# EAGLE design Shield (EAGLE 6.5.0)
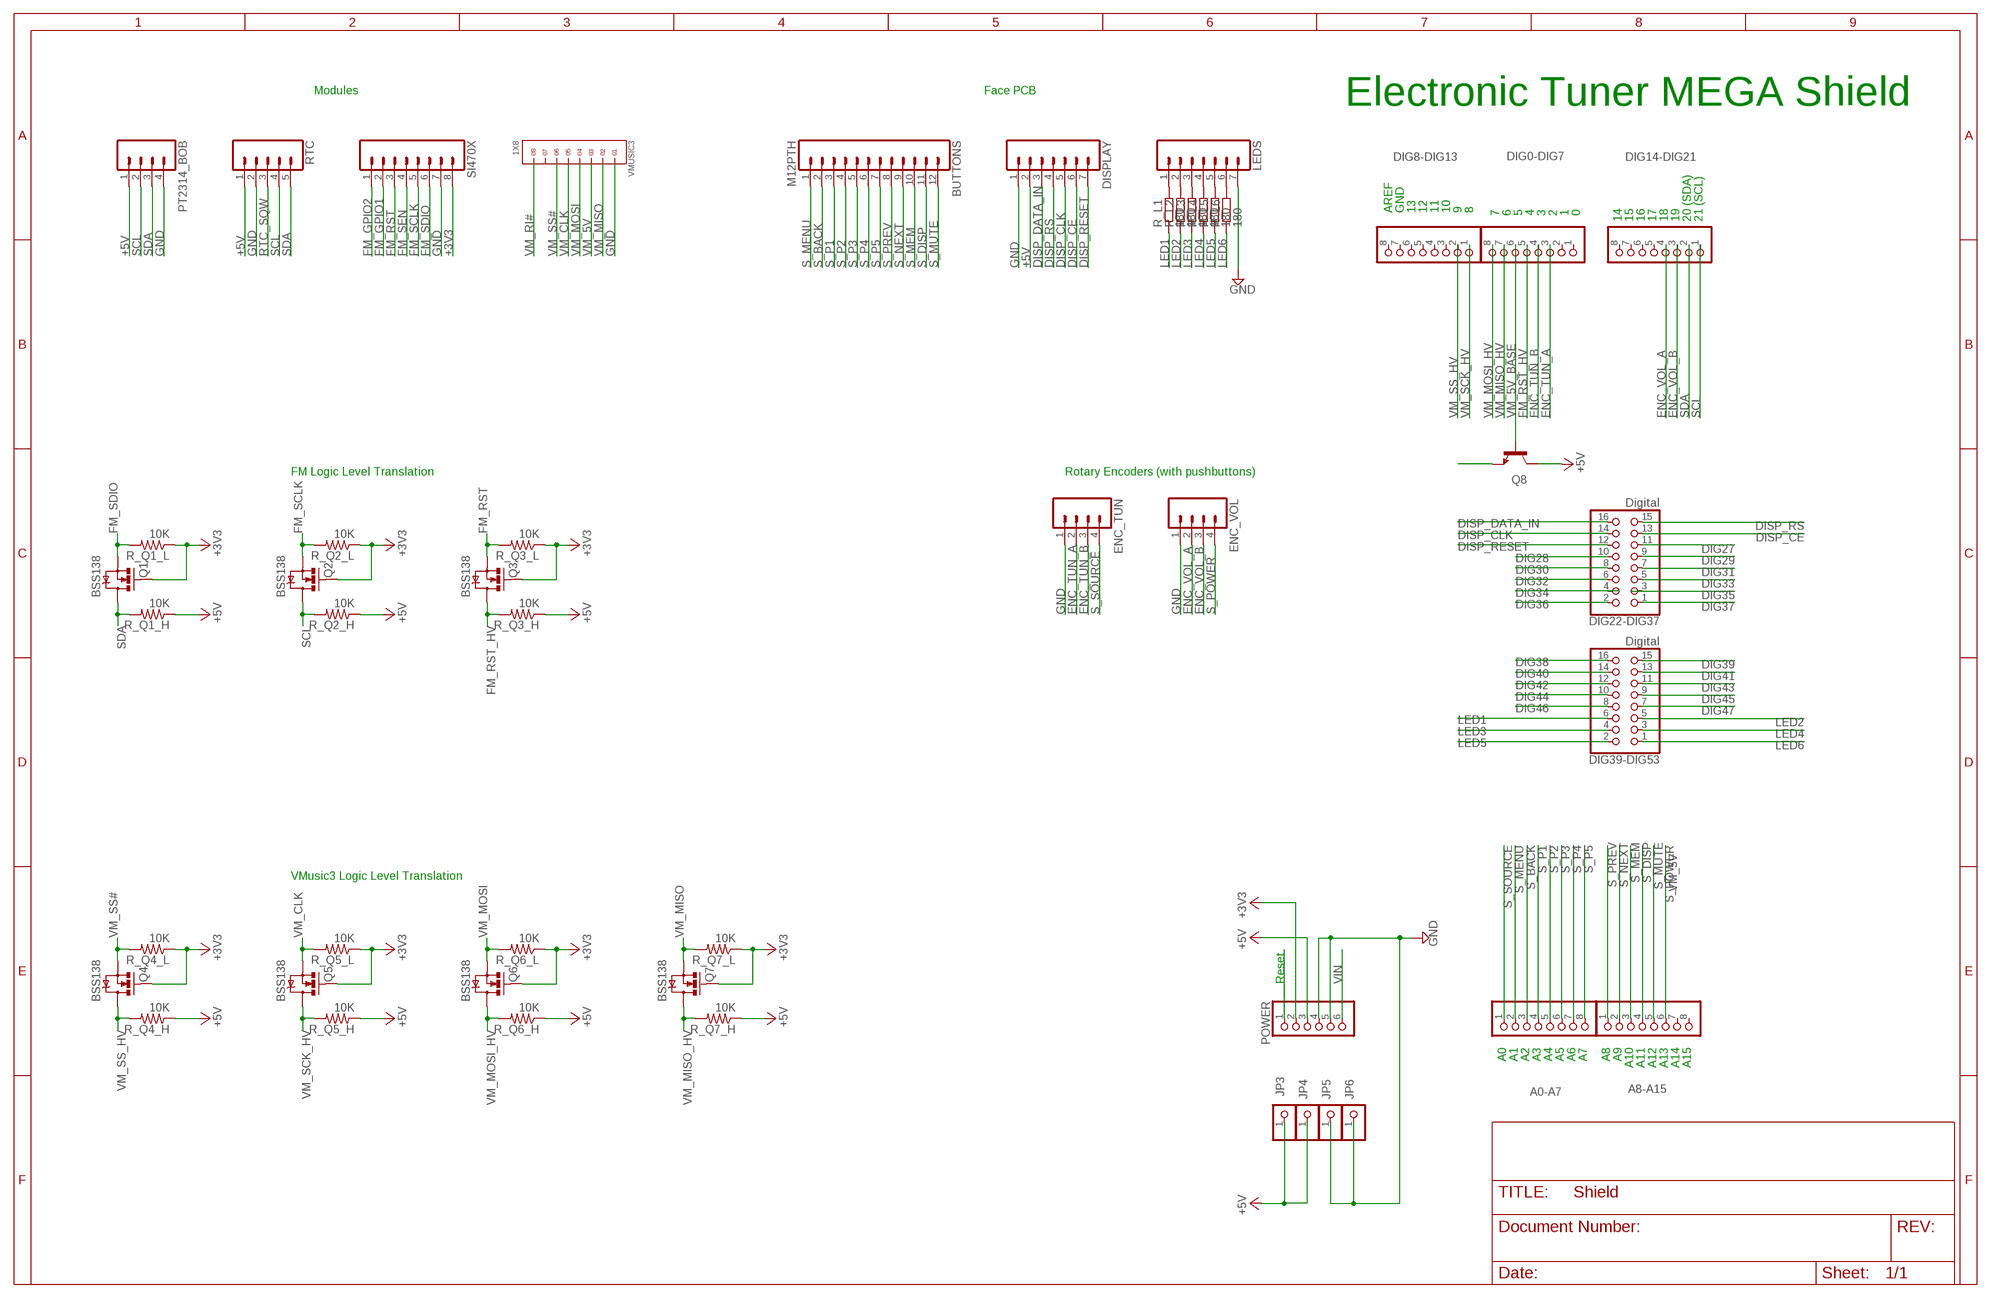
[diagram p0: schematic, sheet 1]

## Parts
A0-A7  PINHD-1X8  [1X08]
A8-A15  PINHD-1X8  [1X08]
BUTTONS  M12PTH  [1X12]
DIG0-DIG7  PINHD-1X8  [1X08]
DIG8-DIG13  PINHD-1X8  [1X08]
DIG14-DIG21  PINHD-1X8  [1X08]
DIG22-DIG37  Digital  PINHD-2X8  [2X08]
DIG39-DIG53  Digital  PINHD-2X8  [2X08]
DISPLAY  M07  [1X07]
ENC_TUN  M04PTH  [1X04]
ENC_VOL  M04PTH  [1X04]
JP3  PINHD-1X1  [1X01]
JP4  PINHD-1X1  [1X01]
JP5  PINHD-1X1  [1X01]
JP6  PINHD-1X1  [1X01]
LEDS  M07  [1X07]
POWER  PINHD-1X6  [1X06]
PT2314_BOB  M04PTH  [1X04]
Q1  BSS138  MOSFET-NCHANNELSMD  [SOT23-3]
Q2  BSS138  MOSFET-NCHANNELSMD  [SOT23-3]
Q3  BSS138  MOSFET-NCHANNELSMD  [SOT23-3]
Q4  BSS138  MOSFET-NCHANNELSMD  [SOT23-3]
Q5  BSS138  MOSFET-NCHANNELSMD  [SOT23-3]
Q6  BSS138  MOSFET-NCHANNELSMD  [SOT23-3]
Q7  BSS138  MOSFET-NCHANNELSMD  [SOT23-3]
Q8  BC848ALT1SMD  [SOT23]
R_L1  180  R-EU_R0603  [R0603]
R_L2  180  R-EU_R0603  [R0603]
R_L3  180  R-EU_R0603  [R0603]
R_L4  180  R-EU_R0603  [R0603]
R_L5  180  R-EU_R0603  [R0603]
R_L6  180  R-EU_R0603  [R0603]
R_Q1_H  10K  RESISTOR0603-RES  [0603-RES]
R_Q1_L  10K  RESISTOR0603-RES  [0603-RES]
R_Q2_H  10K  RESISTOR0603-RES  [0603-RES]
R_Q2_L  10K  RESISTOR0603-RES  [0603-RES]
R_Q3_H  10K  RESISTOR0603-RES  [0603-RES]
R_Q3_L  10K  RESISTOR0603-RES  [0603-RES]
R_Q4_H  10K  RESISTOR0603-RES  [0603-RES]
R_Q4_L  10K  RESISTOR0603-RES  [0603-RES]
R_Q5_H  10K  RESISTOR0603-RES  [0603-RES]
R_Q5_L  10K  RESISTOR0603-RES  [0603-RES]
R_Q6_H  10K  RESISTOR0603-RES  [0603-RES]
R_Q6_L  10K  RESISTOR0603-RES  [0603-RES]
R_Q7_H  10K  RESISTOR0603-RES  [0603-RES]
R_Q7_L  10K  RESISTOR0603-RES  [0603-RES]
RTC  M05PTH  [1X05]
SI470X  M081X08  [1X08]
VMUSIC3  1X8  [1X8]

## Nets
+3V3 [power]: POWER.2 Q1.1(G) Q2.1(G) Q3.1(G) Q4.1(G) Q5.1(G) Q6.1(G) Q7.1(G) R_Q1_L.1 R_Q2_L.1 R_Q3_L.1 R_Q4_L.1 R_Q5_L.1 R_Q6_L.1 R_Q7_L.1 SI470X.8
+5V [power]: DISPLAY.2 JP3.1 JP4.1 POWER.3 PT2314_BOB.1 Q8.3(C) R_Q1_H.1 R_Q2_H.1 R_Q3_H.1 R_Q4_H.1 R_Q5_H.1 R_Q6_H.1 R_Q7_H.1 RTC.1
DIG27: DIG22-DIG37.11
DIG28: DIG22-DIG37.10
DIG29: DIG22-DIG37.9
DIG30: DIG22-DIG37.8
DIG31: DIG22-DIG37.7
DIG32: DIG22-DIG37.6
DIG33: DIG22-DIG37.5
DIG36: DIG22-DIG37.2
DIG37: DIG22-DIG37.1
DIG38: DIG39-DIG53.16
DIG39: DIG39-DIG53.15
DIG40: DIG39-DIG53.14
DIG41: DIG39-DIG53.13
DIG42: DIG39-DIG53.12
DIG43: DIG39-DIG53.11
DIG44: DIG39-DIG53.10
DIG45: DIG39-DIG53.9
DIG46: DIG39-DIG53.8
DIG47: DIG39-DIG53.7
DISP_CE: DIG22-DIG37.13 DISPLAY.6
DISP_CLK: DIG22-DIG37.14 DISPLAY.5
DISP_DATA_IN: DIG22-DIG37.16 DISPLAY.3
DISP_RESET: DIG22-DIG37.12 DISPLAY.7
DISP_RS: DIG22-DIG37.15 DISPLAY.4
ENC_TUN_A: DIG0-DIG7.3 ENC_TUN.2
ENC_TUN_B: DIG0-DIG7.4 ENC_TUN.3
ENC_VOL_A: DIG14-DIG21.4 ENC_VOL.2
ENC_VOL_B: DIG14-DIG21.3 ENC_VOL.3
FM_GPIO1: SI470X.2
FM_GPIO2: SI470X.1
FM_RST: Q3.2(S) R_Q3_L.2 SI470X.3
FM_RST_HV: DIG0-DIG7.5 Q3.3(D) R_Q3_H.2
FM_SCLK: Q2.2(S) R_Q2_L.2 SI470X.5
FM_SDIO: Q1.2(S) R_Q1_L.2 SI470X.6
FM_SEN: SI470X.4
GND [gnd]: DISPLAY.1 ENC_TUN.1 ENC_VOL.1 JP5.1 JP6.1 LEDS.7 POWER.4 POWER.5 PT2314_BOB.4 RTC.2 SI470X.7 VMUSIC3.1
LED1: DIG39-DIG53.6 R_L1.1
LED2: DIG39-DIG53.5 R_L2.1
LED3: DIG39-DIG53.4 R_L3.1
LED4: DIG39-DIG53.3 R_L4.1
LED5: DIG39-DIG53.2 R_L5.1
LED6: DIG39-DIG53.1 R_L6.1
N$13: LEDS.1 R_L1.2
N$14: LEDS.2 R_L2.2
N$15: LEDS.3 R_L3.2
N$16: LEDS.4 R_L4.2
N$17: LEDS.5 R_L5.2
N$18: LEDS.6 R_L6.2
RESET: POWER.1
RTC_SQW: RTC.3
S_BACK: A0-A7.3 BUTTONS.2
S_DISP: A8-A15.4 BUTTONS.11
S_MEM: A8-A15.3 BUTTONS.10
S_MENU: A0-A7.2 BUTTONS.1
S_MUTE: A8-A15.5 BUTTONS.12
S_NEXT: A8-A15.2 BUTTONS.9
S_P1: A0-A7.4 BUTTONS.3
S_P2: A0-A7.5 BUTTONS.4
S_P3: A0-A7.6 BUTTONS.5
S_P4: A0-A7.7 BUTTONS.6
S_P5: A0-A7.8 BUTTONS.7
S_POWER: A8-A15.6 ENC_VOL.4
S_PREV: A8-A15.1 BUTTONS.8
S_SOURCE: A0-A7.1 ENC_TUN.4
SCL: DIG14-DIG21.1 PT2314_BOB.2 Q2.3(D) R_Q2_H.2 RTC.4
SDA: DIG14-DIG21.2 PT2314_BOB.3 Q1.3(D) R_Q1_H.2 RTC.5
VIN [power]: POWER.6
VM_5V [power]: Q8.2(E) VMUSIC3.3
VM_5V_BASE: DIG0-DIG7.6 Q8.1(B)
VM_CLK: Q5.2(S) R_Q5_L.2 VMUSIC3.5
VM_MISO: Q7.2(S) R_Q7_L.2 VMUSIC3.2
VM_MISO_HV: DIG0-DIG7.7 Q7.3(D) R_Q7_H.2
VM_MOSI: Q6.2(S) R_Q6_L.2 VMUSIC3.4
VM_MOSI_HV: DIG0-DIG7.8 Q6.3(D) R_Q6_H.2
VM_RI#: VMUSIC3.8
VM_SCK_HV: DIG8-DIG13.1 Q5.3(D) R_Q5_H.2
VM_SS#: Q4.2(S) R_Q4_L.2 VMUSIC3.6
VM_SS_HV: DIG8-DIG13.2 Q4.3(D) R_Q4_H.2
Unconnected: A8-A15.7 A8-A15.8 DIG0-DIG7.1 DIG0-DIG7.2 DIG8-DIG13.3 DIG8-DIG13.4 DIG8-DIG13.5 DIG8-DIG13.6 DIG8-DIG13.7 DIG8-DIG13.8 DIG14-DIG21.5 DIG14-DIG21.6 DIG14-DIG21.7 DIG14-DIG21.8 DIG22-DIG37.3 DIG22-DIG37.4 VMUSIC3.7

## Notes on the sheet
- Modules | Face PCB
- Electronic Tuner MEGA Shield
- AREF | GND | 13 | 12 | 11 | 10 | 9 | 8 | 7 | 6 | 5 | 4 | 3 | 2 | 1 | 0
- 14 | 15 | 16 | 17 | 18 | 19 | 20 (SDA) | 21 (SCL)
- FM Logic Level Translation | Rotary Encoders (with pushbuttons)
- VMusic3 Logic Level Translation
- Reset
- A0 | A1 | A2 | A3 | A4 | A5 | A6 | A7 | A8 | A9 | A10 | A11 | A12 | A13 | A14 | A15

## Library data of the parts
A0-A7 A8-A15 DIG0-DIG7 DIG8-DIG13 DIG14-DIG21 = pinhead:PINHD-1X8: PIN HEADER
BUTTONS = SparkFun-Connectors:M12: Header 12 Standard 12-pin 0.1" header. Use with straight break away headers (SKU : PRT-00116), right angle break away headers (PRT-00553), swiss pins (PRT-00743), machine pins (PRT-00117), and female headers (PRT-00115).
DIG22-DIG37 DIG39-DIG53 = pinhead:PINHD-2X8: PIN HEADER
DISPLAY LEDS = SparkFun-Connectors:M07: Header 7 Standard 7-pin 0.1" header. Use with straight break away headers (SKU : PRT-00116), right angle break away headers (PRT-00553), swiss pins (PRT-00743), machine pins (PRT-00117), and female headers (PRT-00115). NOTES ON THE VARIANTS LOCK and LOCK_LONGPADS... This footprint was designed to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
ENC_TUN ENC_VOL PT2314_BOB = SparkFun-Connectors:M04: Header 4 Standard 4-pin 0.1" header. Use with straight break away headers (SKU : PRT-00116), right angle break away headers (PRT-00553), swiss pins (PRT-00743), machine pins (PRT-00117), and female headers (PRT-00115). Molex polarized connector foot print use with SKU : PRT-08231 with associated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
JP3-JP6 = pinhead:PINHD-1X1: PIN HEADER
POWER = pinhead:PINHD-1X6: PIN HEADER
Q1-Q7 = SparkFun:MOSFET-NCHANNEL
Q8 = transistor-npn:BC848*: NPN Transistor
R_L1-R_L6 = resistor:R-EU_: RESISTOR, European symbol
R_Q1_H R_Q1_L R_Q2_H R_Q2_L R_Q3_H R_Q3_L R_Q4_H R_Q4_L R_Q5_H R_Q5_L R_Q6_H R_Q6_L R_Q7_H R_Q7_L = SparkFun:RESISTOR: Resistor
RTC = SparkFun-Connectors:M05: Header 5 Standard 5-pin 0.1" header. Use with straight break away headers (SKU : PRT-00116), right angle break away headers (PRT-00553), swiss pins (PRT-00743), machine pins (PRT-00117), and female headers (PRT-00115). Molex polarized connector foot print use with SKU : PRT-08230 with associated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
SI470X = SparkFun-Connectors:M08: Header 8 Standard 8-pin 0.1" header. Use with straight break away headers (SKU : PRT-00116), right angle break away headers (PRT-00553), swiss pins (PRT-00743), machine pins (PRT-00117), and female headers (PRT-00115).
VMUSIC3 = headers(2mm):1X8

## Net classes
0 default: width 0.203 mm, drill 0.406 mm, clearance 0.203 mm
1 power: width 0.61 mm, drill 0.711 mm, clearance 0.203 mm
2 gnd: width 0.305 mm, drill 0.711 mm, clearance 0.203 mm
3 usbvcc: width 0.508 mm, drill 0.711 mm, clearance 0.203 mm

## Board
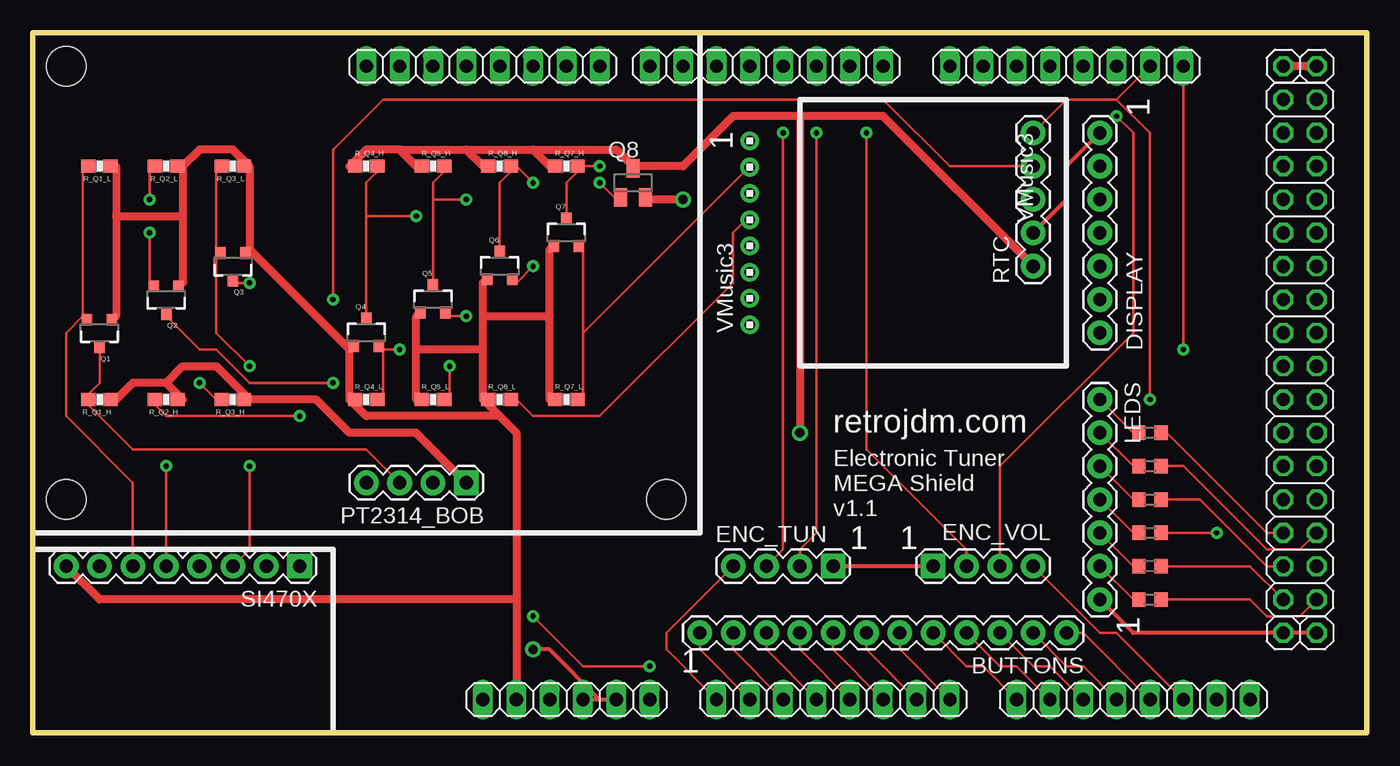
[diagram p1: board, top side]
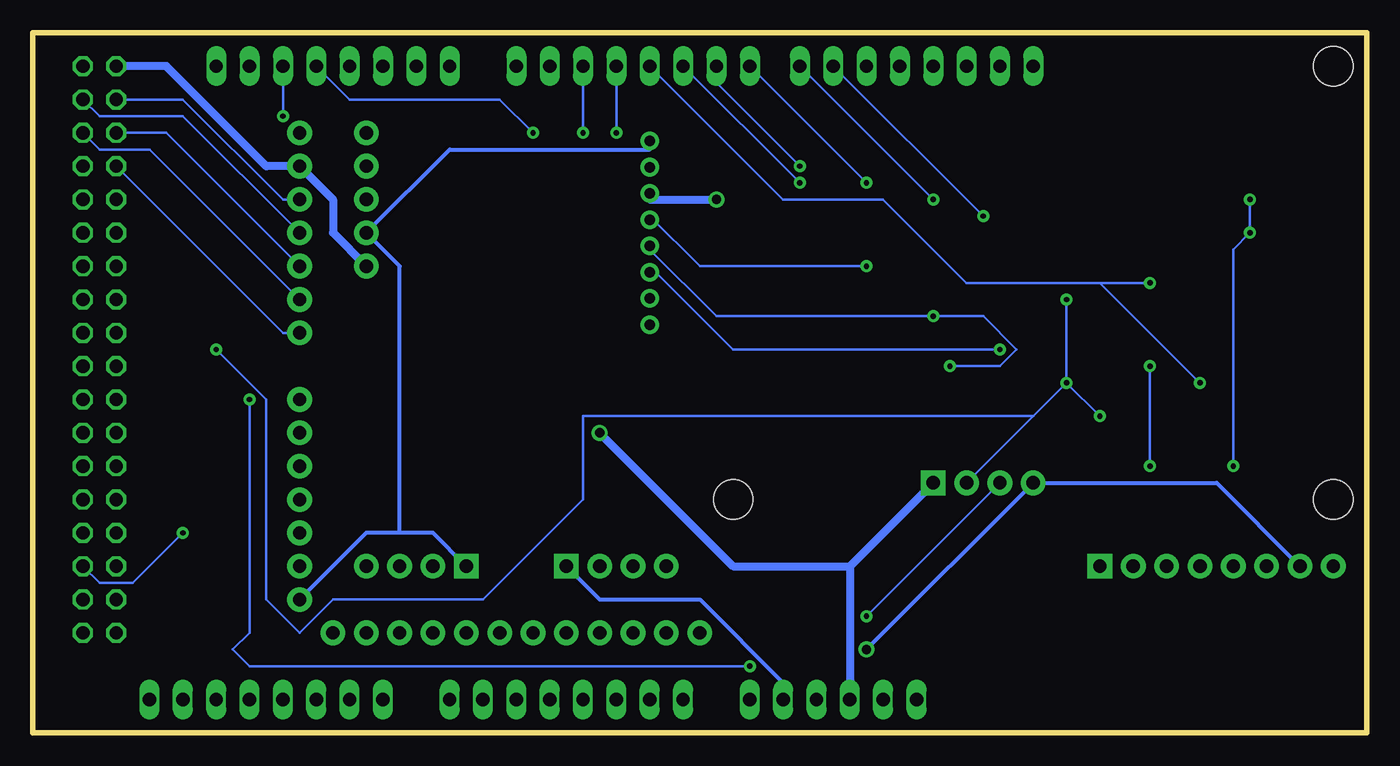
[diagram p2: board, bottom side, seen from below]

Size 101.6 x 53.34 mm. Coordinates in mm from the lower left corner, seen from the top.
Outline: 101.6,53.34 0,53.34 0,0 101.6,0 101.6,53.34
Copper layers (1*16): Top 0.035mm / dielectric 1.5mm / Bottom 0.035mm
Design rules "default *": minimum track width 8mil, minimum drill 16mil, track to track 10mil, track to pad 15mil, pad to pad 15mil, via to via 10mil, smd to smd 10mil, copper to edge 40mil, drill to drill 10mil, minimum pad ring 10mil, minimum via ring 10mil, stop-mask expansion 4mil, vias tented up to drill 0mil, thermal gap 10mil
Holes 3 mm at 48.26,17.78 2.54,17.78 2.54,50.8

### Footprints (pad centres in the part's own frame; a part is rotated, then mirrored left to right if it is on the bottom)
1X08 = drill 1.016 long: 1 -8.89,0; 2 -6.35,0; 3 -3.81,0; 4 -1.27,0; 5 1.27,0; 6 3.81,0; 7 6.35,0; 8 8.89,0
1X12 = drill 1.016 pad 1.88: 1 0,0; 2 2.54,0; 3 5.08,0; 4 7.62,0; 5 10.16,0; 6 12.7,0; 7 15.24,0; 8 17.78,0; 9 20.32,0; 10 22.86,0; 11 25.4,0; 12 27.94,0
2X08 = drill 1.016 octagon: 1 -8.89,-1.27; 2 -8.89,1.27; 3 -6.35,-1.27; 4 -6.35,1.27; 5 -3.81,-1.27; 6 -3.81,1.27; 7 -1.27,-1.27; 8 -1.27,1.27; 9 1.27,-1.27; 10 1.27,1.27; 11 3.81,-1.27; 12 3.81,1.27; 13 6.35,-1.27; 14 6.35,1.27; 15 8.89,-1.27; 16 8.89,1.27
1X07 = drill 1.016 pad 1.88: 1 0,0; 2 2.54,0; 3 5.08,0; 4 7.62,0; 5 10.16,0; 6 12.7,0; 7 15.24,0
1X04 = drill 1.016 pad 1.88 square: 1 0,0 | drill 1.016 pad 1.88: 2 2.54,0; 3 5.08,0; 4 7.62,0
1X01 = drill 1.016 octagon: 1 0,0
1X06 = drill 1.016 long: 1 -6.35,0; 2 -3.81,0; 3 -1.27,0; 4 1.27,0; 5 3.81,0; 6 6.35,0
SOT23-3 = smd 0.8 x 0.9: 1 -0.95,-1; 2 0.95,-1; 3 0,1.1
SOT23 = smd 1 x 1.4: 1 -0.95,-1.1; 2 0.95,-1.1; 3 0,1.1
R0603 = smd 1 x 1.1: 1 -0.85,0; 2 0.85,0
0603-RES = smd 1.1 x 1: 1 -0.85,0; 2 0.85,0
1X05 = drill 1.016 pad 1.88: 1 0,0; 2 2.54,0; 3 5.08,0; 4 7.62,0; 5 10.16,0
1X08' = drill 1.016 pad 1.88 square: 1 0,0 | drill 1.016 pad 1.88: 2 2.54,0; 3 5.08,0; 4 7.62,0; 5 10.16,0; 6 12.7,0; 7 15.24,0; 8 17.78,0
1X8 = drill 0.8 pad 1.422: 1 -7,0; 2 -5,0; 3 -3,0; 4 -1,0; 5 1,0; 6 3,0; 7 5,0; 8 7,0

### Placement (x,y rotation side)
A0-A7  60.96,2.54 0 top
A8-A15  83.82,2.54 0 top
BUTTONS  50.8,7.62 0 top
DIG0-DIG7  55.88,50.8 180 top
DIG8-DIG13  34.29,50.8 180 top
DIG14-DIG21  78.74,50.8 180 top
DIG22-DIG37  96.52,39.37 90 top
DIG39-DIG53  96.52,19.05 90 top
DISPLAY  81.28,45.72 270 top
ENC_TUN  60.96,12.7 180 top
ENC_VOL  68.58,12.7 0 top
JP3  95.25,50.8 0 top
JP4  97.79,50.8 0 top
JP5  95.25,7.62 0 top
JP6  97.79,7.62 0 top
LEDS  81.28,25.4 270 top
POWER  40.64,2.54 0 top
PT2314_BOB  33.02,19.05 180 top
Q1  5.08,30.48 180 top
Q2  10.16,33.02 180 top
Q3  15.24,35.56 180 top
Q4  25.4,30.48 0 top
Q5  30.48,33.02 0 top
Q6  35.56,35.56 0 top
Q7  40.64,38.1 0 top
Q8  45.72,41.91 0 top
R_L1  85.09,22.86 180 top
R_L2  85.09,20.32 180 top
R_L3  85.09,17.78 180 top
R_L4  85.09,15.24 180 top
R_L5  85.09,12.7 180 top
R_L6  85.09,10.16 180 top
R_Q1_H  5.08,25.4 180 top
R_Q1_L  5.08,43.18 180 top
R_Q2_H  10.16,25.4 180 top
R_Q2_L  10.16,43.18 180 top
R_Q3_H  15.24,25.4 180 top
R_Q3_L  15.24,43.18 180 top
R_Q4_H  25.4,43.18 0 top
R_Q4_L  25.4,25.4 0 top
R_Q5_H  30.48,43.18 0 top
R_Q5_L  30.48,25.4 0 top
R_Q6_H  35.56,43.18 0 top
R_Q6_L  35.56,25.4 0 top
R_Q7_H  40.64,43.18 0 top
R_Q7_L  40.64,25.4 0 top
RTC  76.2,35.56 90 top
SI470X  [1X08']  20.32,12.7 180 top
VMUSIC3  54.61,38.1 270 top

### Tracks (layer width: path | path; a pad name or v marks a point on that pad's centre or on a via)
+3V3
  Top 0.61: 11.43,43.18 11.43,39.37 | 11.43,39.37 11.43,34.29 Q2.1 | 6.35,39.37 6.35,43.18 R_Q1_L.1 | 6.35,39.37 6.35,31.75 Q1.1 | 6.35,39.37 11.43,39.37 | 24.13,25.4 24.13,29.21 | 16.51,43.18 16.51,36.83 | 16.51,36.83 24.13,29.21 | 24.13,29.21 Q4.1 | 16.51,36.83 Q3.1 | 11.43,43.18 12.7,44.45 15.24,44.45 16.51,43.18 | 11.43,43.18 R_Q2_L.1 | 16.51,43.18 R_Q3_L.1 | 39.37,31.75 39.37,25.4 R_Q7_L.1 | 39.37,31.75 39.37,36.83 Q7.1 | 29.21,29.21 29.21,25.4 R_Q5_L.1 | 29.21,29.21 29.21,31.75 Q5.1 | 34.29,25.4 34.29,29.21 | 34.29,29.21 34.29,31.75 | 34.29,31.75 34.29,34.29 Q6.1 | 36.83,10.16 36.83,22.86 35.56,24.13 | 36.83,10.16 POWER.2 | 34.29,25.4 35.56,24.13 | 34.29,25.4 R_Q6_L.1 | 34.29,29.21 29.21,29.21 | SI470X.8 5.08,10.16 36.83,10.16 | 34.29,31.75 39.37,31.75 | 24.13,25.4 25.4,24.13 35.56,24.13 | 24.13,25.4 R_Q4_L.1
+5V  (via drill 0.71)
  Top 0.61: 10.16,26.67 7.62,26.67 6.35,25.4 R_Q1_H.1 | 10.16,26.67 11.43,25.4 R_Q2_H.1 | 16.51,25.4 13.97,27.94 11.43,27.94 10.16,26.67 | 16.51,25.4 21.59,25.4 24.13,22.86 29.21,22.86 PT2314_BOB.1 | 16.51,25.4 R_Q3_H.1 | 27.94,44.45 25.4,44.45 24.13,43.18 R_Q4_H.1 | 27.94,44.45 29.21,43.18 R_Q5_H.1 | 33.02,44.45 34.29,43.18 R_Q6_H.1 | 27.94,44.45 33.02,44.45 | 38.1,44.45 39.37,43.18 R_Q7_H.1 | 33.02,44.45 38.1,44.45 | 45.72,43.18 44.45,44.45 38.1,44.45 | JP4.1 JP3.1 | 45.72,43.18 49.53,43.18 53.34,46.99 58.42,46.99 | 58.42,46.99 64.77,46.99 RTC.1 | 45.72,43.18 Q8.3 | 58.42,46.99 v58.42,22.86
  Bottom 0.61: 39.37,12.7 POWER.3 | PT2314_BOB.1 39.37,12.7 | RTC.1 78.74,38.1 78.74,40.64 DISPLAY.2 83.82,43.18 91.44,50.8 JP3.1 | 39.37,12.7 48.26,12.7 v58.42,22.86
DISP_CE
  Bottom 0.203: DIG22-DIG37.13 96.52,44.45 92.71,44.45 DISPLAY.6
DISP_CLK
  Bottom 0.203: DIG22-DIG37.14 91.44,45.72 DISPLAY.5
DISP_DATA_IN
  Bottom 0.203: DIG22-DIG37.16 90.17,48.26 82.55,40.64 DISPLAY.3
DISP_RESET
  Bottom 0.203: DIG22-DIG37.12 82.55,30.48 DISPLAY.7
DISP_RS
  Bottom 0.203: DIG22-DIG37.15 96.52,46.99 90.17,46.99 DISPLAY.4
ENC_TUN_A  (via drill 0.41)
  Top 0.203: v59.69,45.72 59.69,15.24 58.42,13.97 ENC_TUN.2
  Bottom 0.203: v59.69,45.72 DIG0-DIG7.3
ENC_TUN_B  (via drill 0.41)
  Top 0.203: v57.15,45.72 57.15,13.97 ENC_TUN.3
  Bottom 0.203: v57.15,45.72 DIG0-DIG7.4
ENC_VOL_A  (via drill 0.41)
  Top 0.203: v63.5,45.72 63.5,21.59 71.12,13.97 ENC_VOL.2
  Bottom 0.203: DIG14-DIG21.4 77.47,48.26 66.04,48.26 v63.5,45.72
ENC_VOL_B  (via drill 0.41)
  Top 0.203: v82.55,46.99 83.82,45.72 83.82,30.48 73.66,20.32 ENC_VOL.3
  Bottom 0.203: v82.55,46.99 DIG14-DIG21.3
FM_RST  (via drill 0.41)
  Top 0.203: 13.97,36.83 13.97,43.18 R_Q3_L.2 | 13.97,36.83 13.97,30.48 v16.51,27.94 | v16.51,20.32 16.51,13.97 SI470X.3 | 13.97,36.83 Q3.2
  Bottom 0.203: v16.51,20.32 v16.51,27.94
FM_RST_HV  (via drill 0.41)
  Top 0.203: v16.51,34.29 15.24,34.29 Q3.3 | v12.7,26.67 13.97,25.4 R_Q3_H.2
  Bottom 0.203: 20.32,34.29 30.48,34.29 36.83,40.64 44.45,40.64 DIG0-DIG7.5 | 20.32,34.29 v16.51,34.29 | 20.32,34.29 v12.7,26.67
FM_SCLK  (via drill 0.41)
  Top 0.203: v8.89,38.1 8.89,34.29 Q2.2 | v8.89,40.64 8.89,43.18 R_Q2_L.2 | v10.16,20.32 SI470X.5
  Bottom 0.203: v8.89,40.64 v8.89,38.1 10.16,36.83 v10.16,20.32
FM_SDIO
  Top 0.203: 3.81,31.75 3.81,43.18 R_Q1_L.2 | SI470X.6 7.62,19.05 2.54,24.13 2.54,30.48 3.81,31.75 | 3.81,31.75 Q1.2
GND  (via drill 0.71)
  Top 0.305: DISPLAY.1 78.74,43.18 78.74,40.64 RTC.2 | JP6.1 JP5.1 83.82,7.62 LEDS.7 | POWER.5 43.18,2.54 | 43.18,2.54 POWER.4 | ENC_VOL.1 ENC_TUN.1 | v38.1,6.35 39.37,6.35 43.18,2.54
  Bottom 0.305: VMUSIC3.1 54.61,44.45 69.85,44.45 RTC.2 73.66,35.56 73.66,15.24 | SI470X.7 11.43,19.05 PT2314_BOB.4 v38.1,6.35 | POWER.5 44.45,3.81 50.8,10.16 58.42,10.16 ENC_TUN.1 | LEDS.7 76.2,15.24 73.66,15.24 | 73.66,15.24 71.12,15.24 ENC_VOL.1
LED1
  Top 0.203: DIG39-DIG53.6 93.98,15.24 86.36,22.86 R_L1.1
LED2
  Top 0.203: R_L2.1 87.63,20.32 93.98,13.97 96.52,13.97 DIG39-DIG53.5
LED3
  Top 0.203: R_L3.1 88.9,17.78 93.98,12.7 DIG39-DIG53.4
LED4  (via drill 0.41)
  Top 0.203: v90.17,15.24 R_L4.1
  Bottom 0.203: v90.17,15.24 93.98,11.43 96.52,11.43 DIG39-DIG53.3
LED5
  Top 0.203: R_L5.1 92.71,12.7 DIG39-DIG53.2
LED6
  Top 0.203: R_L6.1 92.71,10.16 93.98,8.89 96.52,8.89 DIG39-DIG53.1
N$13
  Top 0.203: LEDS.1 83.82,22.86 R_L1.2
N$14
  Top 0.203: LEDS.2 83.82,20.32 R_L2.2
N$15
  Top 0.203: LEDS.3 83.82,17.78 R_L3.2
N$16
  Top 0.203: LEDS.4 83.82,15.24 R_L4.2
N$17
  Top 0.203: LEDS.5 83.82,12.7 R_L5.2
N$18
  Top 0.203: LEDS.6 83.82,10.16 R_L6.2
S_BACK
  Top 0.203: A0-A7.3 53.34,6.35 BUTTONS.2
S_DISP
  Top 0.203: A8-A15.4 80.01,5.08 78.74,5.08 BUTTONS.11
S_MEM
  Top 0.203: A8-A15.3 77.47,5.08 76.2,5.08 BUTTONS.10
S_MENU
  Top 0.203: A0-A7.2 50.8,6.35 BUTTONS.1
S_MUTE
  Top 0.203: A8-A15.5 80.01,7.62 BUTTONS.12
S_NEXT
  Top 0.203: A8-A15.2 74.93,5.08 73.66,5.08 BUTTONS.9
S_P1
  Top 0.203: A0-A7.4 55.88,6.35 BUTTONS.3
S_P2
  Top 0.203: A0-A7.5 58.42,6.35 BUTTONS.4
S_P3
  Top 0.203: A0-A7.6 60.96,6.35 BUTTONS.5
S_P4
  Top 0.203: A0-A7.7 63.5,6.35 BUTTONS.6
S_P5
  Top 0.203: A0-A7.8 66.04,6.35 BUTTONS.7
S_POWER
  Top 0.203: A8-A15.6 82.55,7.62 81.28,7.62 ENC_VOL.4
S_PREV
  Top 0.203: A8-A15.1 72.39,5.08 71.12,5.08 BUTTONS.8
S_SOURCE
  Top 0.203: A0-A7.1 48.26,6.35 48.26,7.62 ENC_TUN.4
SCL  (via drill 0.41)
  Top 0.203: v22.86,26.67 16.51,26.67 13.97,29.21 12.7,29.21 10.16,31.75 Q2.3 | v20.32,24.13 10.16,24.13 8.89,25.4 R_Q2_H.2 | v87.63,29.21 DIG14-DIG21.1 | RTC.4 69.85,43.18 64.77,48.26 26.67,48.26 22.86,44.45 v22.86,33.02
  Bottom 0.203: PT2314_BOB.2 25.4,24.13 | 25.4,24.13 v22.86,26.67 | v22.86,26.67 v20.32,24.13 | v87.63,29.21 83.82,25.4 83.82,10.16 81.28,7.62 78.74,10.16 67.31,10.16 59.69,17.78 59.69,24.13 25.4,24.13 | v22.86,26.67 v22.86,33.02
SDA  (via drill 0.41)
  Top 0.203: 82.55,48.26 DIG14-DIG21.2 | 82.55,48.26 78.74,48.26 RTC.5 | Q1.3 5.08,26.67 3.81,25.4 | 3.81,25.4 7.62,21.59 25.4,21.59 PT2314_BOB.3 | 3.81,25.4 R_Q1_H.2 | 82.55,48.26 85.09,45.72 v85.09,25.4 | v46.99,5.08 41.91,5.08 v38.1,8.89
  Bottom 0.203: v85.09,25.4 85.09,7.62 86.36,6.35 85.09,5.08 v46.99,5.08 | PT2314_BOB.3 v38.1,8.89
VM_5V  (via drill 0.71)
  Top 0.61: v49.53,40.64 46.99,40.64 Q8.2
  Bottom 0.61: v49.53,40.64 54.61,40.64 VMUSIC3.3
VM_5V_BASE  (via drill 0.41)
  Top 0.203: v43.18,41.91 44.45,40.64 Q8.1
  Bottom 0.203: DIG0-DIG7.6 v43.18,41.91
VM_CLK  (via drill 0.41)
  Top 0.203: v33.02,31.75 31.75,31.75 Q5.2 | v31.75,27.94 31.75,25.4 R_Q5_L.2
  Bottom 0.203: VMUSIC3.5 54.61,36.83 49.53,31.75 v33.02,31.75 29.21,31.75 26.67,29.21 27.94,27.94 v31.75,27.94
VM_MISO
  Top 0.203: 41.91,30.48 41.91,25.4 R_Q7_L.2 | 41.91,30.48 41.91,36.83 Q7.2 | 41.91,30.48 54.61,43.18 VMUSIC3.2
VM_MISO_HV  (via drill 0.41)
  Top 0.203: Q7.3 40.64,41.91 41.91,43.18 | v43.18,43.18 41.91,43.18 | 41.91,43.18 R_Q7_H.2
  Bottom 0.203: v43.18,43.18 49.53,49.53 DIG0-DIG7.7
VM_MOSI  (via drill 0.41)
  Top 0.203: v38.1,35.56 36.83,34.29 Q6.2 | R_Q6_L.2 36.83,25.4 38.1,24.13 43.18,24.13 53.34,34.29 53.34,38.1 54.61,39.37 VMUSIC3.4
  Bottom 0.203: v38.1,35.56 50.8,35.56 54.61,39.37 VMUSIC3.4
VM_MOSI_HV  (via drill 0.41)
  Top 0.203: Q6.3 35.56,41.91 36.83,43.18 | 36.83,43.18 v38.1,41.91 | 36.83,43.18 R_Q6_H.2
  Bottom 0.203: v38.1,41.91 DIG0-DIG7.8
VM_SCK_HV  (via drill 0.41)
  Top 0.203: 30.48,40.64 30.48,41.91 31.75,43.18 R_Q5_H.2 | 30.48,40.64 Q5.3 | 30.48,40.64 v33.02,40.64
  Bottom 0.203: v33.02,40.64 DIG8-DIG13.1
VM_SS#  (via drill 0.41)
  Top 0.203: 26.67,29.21 26.67,25.4 R_Q4_L.2 | v27.94,29.21 26.67,29.21 | 26.67,29.21 Q4.2
  Bottom 0.203: v27.94,29.21 48.26,29.21 54.61,35.56 VMUSIC3.6
VM_SS_HV  (via drill 0.41)
  Top 0.203: 25.4,39.37 25.4,41.91 26.67,43.18 R_Q4_H.2 | 25.4,39.37 Q4.3 | 25.4,39.37 v29.21,39.37
  Bottom 0.203: v29.21,39.37 DIG8-DIG13.2

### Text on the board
tNames: 1 | VMusic3 | 1 | VMusic3 | retrojdm.com | Electronic Tuner / MEGA Shield / v1.1 | 1 | 1 | 1 | 1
